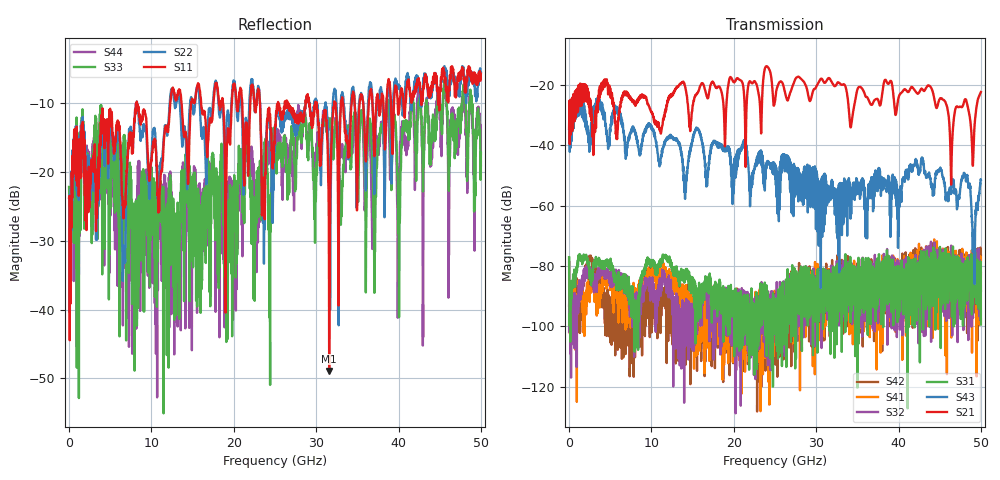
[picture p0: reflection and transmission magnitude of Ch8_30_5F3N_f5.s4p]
!Agilent Technologies,N5247A,US51170199,A.09.90.13
!Agilent N5247A: A.09.90.13
!Date: Wednesday, December 16, 2015 10:26:56
!Correction: S11(Full 4 Port(1,2,3,4))
!S12(Full 4 Port(1,2,3,4))
!S13(Full 4 Port(1,2,3,4))
!S14(Full 4 Port(1,2,3,4))
!S21(Full 4 Port(1,2,3,4))
!S22(Full 4 Port(1,2,3,4))
!S23(Full 4 Port(1,2,3,4))
!S24(Full 4 Port(1,2,3,4))
!S31(Full 4 Port(1,2,3,4))
!S32(Full 4 Port(1,2,3,4))
!S33(Full 4 Port(1,2,3,4))
!S34(Full 4 Port(1,2,3,4))
!S41(Full 4 Port(1,2,3,4))
!S42(Full 4 Port(1,2,3,4))
!S43(Full 4 Port(1,2,3,4))
!S44(Full 4 Port(1,2,3,4))
!S4P File: Measurements: <S11,S12,S13,S14>,
!<S21,S22,S23,S24>,
!<S31,S32,S33,S34>,
!<S41,S42,S43,S44>:
# Hz S  dB  R 50
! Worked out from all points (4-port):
!   3201 points, 10 MHz to 50 GHz, reference 50 ohm
!   strongest paths, dB at 10 MHz, 12.51 GHz, 25 GHz, 37.5 GHz, 50 GHz:
!     S21: -34.4, -23.5, -25.4, -24.8, -22.3
!     S43: -34.5, -37.3, -46.9, -48.5, -51.4
!     S31: -77.0, -80.8, -95.8, -84.1, -99.3
!     S32: -101.7, -90.6, -94.2, -96.7, -88.1
!     S41: -93.1, -86.2, -94.2, -82.1, -82.2
!     S42: -77.3, -93.5, -95.4, -89.2, -76.5
!   lowest |S11| = -48.9 dB at 31.58 GHz (marker M1), VSWR 1.01, Z = 50.3 + j0.107 ohm
!   |S11| at or under -10 dB: start of sweep to 8.215 GHz; 8.249 GHz to 12.28 GHz (4.028 GHz wide, 39.2 % of centre); 23.18 GHz to 25.36 GHz (2.175 GHz wide, 8.96 % of centre)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
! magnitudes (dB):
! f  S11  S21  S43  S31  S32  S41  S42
! 10 MHz  -23.7  -34.4  -34.5  -77.0  -101.7  -93.1  -77.3
! 14.13 GHz  -14.2  -21.2  -51.6  -82.6  -106.5  -92.5  -112.8
! 15.66 GHz  -7.1  -22.3  -34.7  -89.7  -92.5  -101.6  -95.2
! 31.58 GHz  -48.9  -17.7  -56.5  -89.8  -93.9  -83.0  -89.7
! 46.41 GHz  -5.1  -50.2  -55.3  -82.5  -81.0  -103.6  -93.4
! 49.13 GHz  -6.9  -38.9  -71.0  -87.8  -88.1  -80.0  -83.8
! 50 GHz  -5.7  -22.3  -51.4  -99.3  -88.1  -82.2  -76.5
